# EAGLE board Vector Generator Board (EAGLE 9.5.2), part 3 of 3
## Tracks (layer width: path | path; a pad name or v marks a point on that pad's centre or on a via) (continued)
VRAM3  (via drill 0.35) (continued)
  Bottom 0.381: v4.36,171.92 4.65,171.92 4.65,170.46 P1.6 | v80.01,65.89 56.06,65.89 52.55,62.38 38.24,62.38 37.07,61.21 1G.5 | v80.89,94.81 79.43,96.27 79.43,97.73 75.34,97.73 v74.46,98.6 | v74.46,125.77 74.17,126.06 71.25,126.06 v67.45,129.86 | v67.45,153.52 67.16,153.81 60.44,153.81 58.1,156.15 38.24,156.15 37.07,157.31 1D.9 | v24.8,157.61 v10.49,157.61
VRAM4  (via drill 0.35)
  Top 0.381: v4.94,168.12 4.94,166.66 P1.7 4.94,166.37 7.28,164.03 9.61,164.03 v9.61,156.44 | v34.44,76.99 34.44,101.52 35.03,102.11 | 35.03,102.11 36.78,103.86 1F.2 | 52.84,151.18 52.84,133.07 52.26,132.49 52.26,98.02 v52.55,97.73 | 52.84,151.18 v52.84,235.01 | 35.03,102.11 v35.03,100.36 | v24.8,156.44 30.06,151.18 v31.23,151.18 | 52.84,151.18 v53.14,151.18
  Bottom 0.381: v4.94,168.12 4.94,166.66 P1.7 | v34.44,76.99 31.52,76.99 31.52,63.84 36.78,58.59 1G.6 | v52.84,235.01 38.24,235.01 37.07,236.18 1B.6 | v52.55,97.73 40.58,97.73 37.95,100.36 v35.03,100.36 | v24.8,156.44 v9.61,156.44 | v53.14,151.18 v31.23,151.18
VRAM5  (via drill 0.35)
  Top 0.381: v46.42,57.12 46.42,79.62 42.62,83.41 42.62,84.29 43.5,85.17 47.59,85.17 47.59,91.88 48.17,92.47 48.17,100.06 v47.88,100.36 | v32.11,233.55 31.81,233.26 31.81,225.37 v24.8,218.36 | v19.84,181.56 v19.84,216.03 | v4.94,164.03 4.94,162.57 P1.8 | v24.8,105.91 24.8,108.24 32.69,108.24 34.15,106.78 34.15,105.61 37.66,105.61 38.82,104.44 38.82,103.57 37.07,101.82 1F.3 | v11.07,105.91 10.78,106.2 10.78,140.08 12.24,141.54 v12.24,162.57
  Bottom 0.381: v46.42,57.12 38.24,57.12 37.07,55.96 1G.7 | v47.88,100.36 38.82,100.36 37.66,101.52 37.07,101.52 1F.3 | v32.11,233.55 36.78,233.55 1B.7 | v24.8,218.36 22.47,216.03 v19.84,216.03 | v19.84,181.56 11.07,172.8 10.2,172.8 9.61,172.21 9.61,164.03 | 9.61,162.57 9.61,164.03 | 9.61,162.57 4.94,162.57 P1.8 | 9.61,164.03 v4.94,164.03 | v11.07,105.91 v24.8,105.91 | 9.61,162.57 v12.24,162.57
VRAM6  (via drill 0.35)
  Top 0.381: v49.34,54.5 49.34,81.66 48.17,82.83 48.17,91.59 48.75,92.18 48.75,102.4 v48.46,102.69 | v35.03,204.93 35.03,213.98 37.36,216.32 37.36,218.36 35.03,220.7 35.03,229.17 36.78,230.92 1B.8 | v35.03,202.3 35.03,182.44 36.78,180.68 36.78,180.1 32.98,176.3 v32.98,164.03 32.98,163.16 28.6,158.78 v24.8,158.78 | v4.94,160.24 4.94,158.78 P1.9 | v58.69,102.69 58.98,102.98 58.98,116.42 58.1,117.3 58.1,121.97 58.98,122.85 58.98,123.72 58.1,124.6 55.18,124.6 v55.18,150.31 | v51.38,150.31 51.09,150.6 51.09,163.74 v51.38,164.03
  Bottom 0.381: v49.34,54.5 37.95,54.5 37.07,53.62 1G.8 | 1F.4 36.78,99.19 34.15,99.19 34.15,101.23 35.61,102.69 v48.46,102.69 v58.69,102.69 | v35.03,202.3 v35.03,204.93 | 4.94,158.78 v24.8,158.78 | 4.94,158.78 v4.94,160.24 | 4.94,158.78 P1.9 | v51.38,150.31 v55.18,150.31 | v32.98,164.03 v51.38,164.03
VRAM7  (via drill 0.35)
  Top 0.381: v4.94,156.15 4.94,154.69 P1.10 | 1G.9 36.78,50.99 35.03,52.74 35.03,72.9 36.78,74.65 36.78,81.66 35.03,83.41 35.03,94.51 36.78,96.27 1F.5 | v42.33,228.59 42.62,228.29 42.62,217.49 47.59,212.52 47.59,185.65 48.46,184.77 48.46,182.44 49.05,181.85 49.05,167.83 48.75,167.54 48.75,150.01 | 48.75,150.01 48.75,135.41 47,133.66 47,128.4 47.3,128.11 47.3,127.52 47,127.23 47,93.05 v47.3,92.76 | v24.8,154.39 25.97,154.39 30.35,150.01 v31.23,150.01 | 48.75,150.01 v48.46,150.01
  Bottom 0.381: v4.94,156.15 4.94,154.69 P1.10 4.94,154.39 v24.8,154.39 | v42.33,228.59 37.07,228.59 1B.9 | v47.3,92.76 40.58,92.76 37.07,96.27 1F.5 | v48.46,150.01 v31.23,150.01
VRAM8  (via drill 0.35)
  Top 0.381: 1F.6 39.41,96.56 39.41,106.78 35.9,110.29 20.13,110.29 v20.13,140.96 | v32.11,210.77 32.11,194.41 22.76,185.06 v22.76,181.56 | v19.84,143.59 v19.84,179.22 | v4.94,148.84 4.94,150.31 P1.11
  Bottom 0.381: 17.5,143.59 10.78,150.31 4.94,150.31 | 17.5,143.59 v20.13,140.96 | v32.11,210.77 36.78,210.77 1C.2 | v22.76,181.56 20.42,179.22 v19.84,179.22 | 17.5,143.59 v19.84,143.59 | 4.94,150.31 v4.94,148.84 | 4.94,150.31 P1.11
VRAM9  (via drill 0.35)
  Top 0.381: v31.23,111.16 28.89,113.5 21.3,113.5 v21.3,140.08 | v31.23,208.14 31.52,207.85 31.52,194.7 21.59,184.77 v21.59,181.56 | v21.01,143.59 v21.01,178.35 | v4.94,145.05 4.94,146.51 P1.12
  Bottom 0.381: v31.23,111.16 30.94,111.16 30.94,97.43 36.78,91.59 1F.7 | 21.01,140.08 14.58,140.08 9.61,145.05 | 9.61,145.05 8.15,146.51 4.94,146.51 P1.12 | v31.23,208.14 36.78,208.14 1C.3 | v21.59,181.56 20.13,180.1 19.55,180.1 18.96,179.51 18.96,178.35 v21.01,178.35 | 21.01,140.08 v21.01,143.59 | 21.01,140.08 v21.3,140.08 | 9.61,145.05 v4.94,145.05
VRAM10  (via drill 0.35)
  Top 0.381: v49.05,90.13 49.34,90.42 49.34,114.38 v49.05,114.67 | v31.23,115.25 23.05,123.43 v23.05,137.74 | 9.61,139.79 v9.61,137.74 | 9.61,139.79 6.98,142.42 4.94,142.42 P1.13 | v24.8,183.6 24.8,184.77 33.27,193.24 33.27,203.76 35.03,203.76 36.78,205.51 1C.4 | 11.37,142.42 11.37,141.54 9.61,139.79 | 11.37,142.42 v11.37,183.6 | 11.37,142.42 v11.07,142.42
  Bottom 0.381: v49.05,90.13 38.24,90.13 37.07,88.96 1F.8 | v49.05,114.67 48.75,114.96 31.52,114.96 v31.23,115.25 | v9.61,137.74 v23.05,137.74 | v11.37,183.6 v24.8,183.6 | v11.07,142.42 4.94,142.42 P1.13
VRAM11  (via drill 0.35)
  Top 0.381: v41.16,118.17 v41.16,86.34 | v31.23,118.17 23.93,125.48 v23.93,138.62 | v34.15,181.56 34.15,203.18 36.78,203.18 1C.5 | v31.23,179.22 24.8,172.8 23.93,172.8 v23.93,144.46 | v4.94,140.37 4.94,138.91 P1.14
  Bottom 0.381: v41.16,86.34 37.07,86.34 1F.9 | v31.23,118.17 v41.16,118.17 | 22.17,138.62 4.94,138.62 P1.14 4.94,138.91 v4.94,140.37 | 22.17,138.62 v23.93,138.62 | v34.15,181.56 31.81,179.22 v31.23,179.22 | v23.93,144.46 22.76,144.46 22.17,143.88 22.17,138.62
VRAMPC  (via drill 0.35)
  Top 0.381: v12.54,118.76 12.54,38.14 22.76,38.14 31.81,29.08 31.81,19.44 34.73,19.44 35.32,20.03 35.32,20.61 35.03,20.9 35.03,24.7 36.78,26.45 1H.3 | v4.94,120.51 4.94,119.05 P1.19
  Bottom 0.381: v12.54,118.76 4.94,118.76 P1.19 4.94,119.05 v4.94,120.51
XBRM1
  Top 0.381: 4A.13 105.42,277.95 115.65,267.73 115.65,251.08 120.03,246.7 120.03,240.56 118.28,238.81 5B.4
XBRM2
  Top 0.381: 4A.12 105.42,275.32 115.06,265.68 115.06,249.33 117.98,246.41 5B.1
XBRM3  (via drill 0.35)
  Top 0.381: v128.5,272.99 v128.5,241.44
  Bottom 0.381: v128.5,241.44 125.87,241.44 5B.14 | v128.5,272.99 105.42,272.99 4A.11
XBRM4  (via drill 0.35)
  Top 0.381: v103.38,245.24 103.67,245.53 103.67,268.9 105.13,270.36 4A.10 | v123.24,270.36 123.24,246.41 125.58,244.07 5B.15
  Bottom 0.381: v103.38,245.24 97.83,245.24 4B.1 | v123.24,270.36 105.42,270.36 4A.10
XBRM5
  Bottom 0.381: 4B.13 105.42,242.61 105.72,242.9 116.52,242.9 117.4,243.78 117.98,243.78 5B.2
XBRM6
  Bottom 0.381: 4B.12 105.42,240.27 106.01,240.86 117.69,240.86 117.98,241.15 5B.3
XBRM7  (via drill 0.35)
  Top 0.381: v102.5,274.15 102.5,240.27 105.13,237.64 4B.11
  Bottom 0.381: v102.5,274.15 117.98,274.15 5A.4
XBRM8  (via drill 0.35)
  Top 0.381: v103.38,209.6 103.67,209.89 103.67,215.74 106.59,218.66 106.59,228.88 107.17,229.46 107.17,232.97 105.42,234.72 4B.10 | v120.61,235.01 120.61,246.99 116.23,251.37 116.23,280 117.98,281.75 5A.1
  Bottom 0.381: v103.38,209.6 97.83,209.6 4C.1 | v120.61,235.01 105.42,235.01 4B.10
XBRM9  (via drill 0.35)
  Top 0.381: v99.87,207.26 99.87,266.85 100.17,267.14 v100.17,279.41
  Bottom 0.381: v99.87,207.26 105.13,207.26 4C.13 | v100.17,279.41 115.94,279.41 117.11,280.58 122.07,280.58 125.58,277.08 5A.14
XBRM10  (via drill 0.35)
  Top 0.381: v140.18,208.14 140.18,222.75 135.22,227.71 135.22,270.65 126.75,279.12 125.87,279.12 5A.15
  Bottom 0.381: v140.18,208.14 136.97,208.14 133.46,204.63 105.42,204.63 4C.12
XBRM11  (via drill 0.35)
  Top 0.381: v101.33,202.01 101.62,202.3 101.62,215.44 102.79,216.61 102.79,239.1 101.62,240.27 v101.62,277.08
  Bottom 0.381: v101.33,202.01 105.13,202.01 4C.11 | v101.62,277.08 115.94,277.08 117.98,279.12 5A.2
XBRM12  (via drill 0.35)
  Top 0.381: v112.43,198.79 112.73,199.09 112.73,215.44 113.02,215.74 113.02,223.62 | 113.02,223.62 113.02,239.4 111.56,240.86 111.56,268.31 108.05,271.82 103.67,271.82 103.67,278.83 104.25,279.41 108.34,279.41 v108.34,276.2 | v221.68,220.99 221.68,206.39 219.93,204.63 10C.3 | v99,223.62 v99,220.99 | 113.02,223.62 v112.73,223.62
  Bottom 0.381: 4C.10 106.01,198.79 v112.43,198.79 | v108.34,276.2 108.64,276.49 117.69,276.49 117.98,276.78 5A.3 | v221.68,220.99 159.46,220.99 159.17,221.28 142.81,221.28 142.52,220.99 112.14,220.99 111.85,221.28 102.21,221.28 101.92,220.99 v99,220.99 | v112.73,223.62 v99,223.62
XBRMCLK  (via drill 0.35)
  Top 0.381: 5B.9 125.87,228.88 127.62,230.63 127.62,262.18 125.87,263.93 5A.9 | v134.34,228.59 134.34,227.71 136.09,225.96 136.09,203.18 144.86,203.18 146.03,204.34 6C.12
  Bottom 0.381: v134.34,228.59 125.87,228.59 5B.9
XEND1  (via drill 0.35)
  Top 0.381: v58.98,263.06 58.98,248.16 57.23,246.41 2B.2 | v132.59,257.5 v132.59,208.43 | v186.63,257.5 186.63,263.93 8A.9 | v83.22,259.26 83.22,264.81 84.98,266.56 3A.10
  Bottom 0.381: 1B.19 44.67,246.41 56.93,246.41 2B.2 | v58.98,263.06 81.47,263.06 84.98,266.56 3A.10 | v132.59,208.43 125.87,208.43 5C.15 | v186.63,257.5 132.88,257.5 | v83.22,259.26 131.13,259.26 132.88,257.5 | 132.88,257.5 v132.59,257.5
XEND2  (via drill 0.35)
  Top 0.381: v77.67,255.75 77.67,263.93 3A.8 | 5C.1 118.28,210.77 121.49,207.56 123.83,207.56 123.83,234.72 121.2,237.35 v121.2,255.75 v121.2,265.39 | v59.86,255.75 59.86,246.7 57.23,244.07 2B.3
  Bottom 0.381: 1B.18 44.67,243.78 56.93,243.78 2B.3 | v121.2,255.75 v77.67,255.75 v59.86,255.75 | v121.2,265.39 146.9,265.39 148.07,266.56 167.35,266.56 168.81,268.02 185.46,268.02 186.63,269.19 8A.11
XEND3  (via drill 0.35)
  Top 0.381: v123.83,197.04 124.12,197.04 125.58,195.58 5C.10 | v91.4,220.99 v91.4,198.21 | v69.79,220.99 v69.79,239.98 69.79,271.82 v70.08,272.11 | 75.34,274.74 74.17,273.57 v74.17,272.11 | 75.34,274.74 77.38,276.78 3A.3 | v188.67,289.64 188.67,278.83 186.92,277.08 8A.14 | 75.34,274.74 v75.34,289.64
  Bottom 0.381: v123.83,197.04 107.47,197.04 106.3,198.21 v91.4,198.21 | v69.79,220.99 v91.4,220.99 | v69.79,239.98 58.39,239.98 57.23,241.15 2B.4 56.93,241.44 44.67,241.44 1B.17 | v70.08,272.11 v74.17,272.11 | v75.34,289.64 v188.67,289.64
XEND4  (via drill 0.35)
  Top 0.381: 74.46,290.51 64.82,290.51 64.82,282.63 63.94,281.75 61.61,281.75 61.61,243.19 57.23,238.81 2B.5 | 74.46,290.51 75.63,290.51 76.21,289.93 76.21,283.21 77.38,282.04 3A.1 | v170.56,278.54 v170.56,193.24 | v74.46,289.05 74.46,290.51 | v179.03,288.76 179.03,282.04 8A.1
  Bottom 0.381: 1B.16 44.67,238.81 56.93,238.81 2B.5 | v170.56,193.24 169.98,192.66 164.72,192.66 161.8,195.58 157.71,195.58 155.37,193.24 144.86,193.24 142.52,195.58 137.26,195.58 135.51,193.83 126.45,193.83 125.87,193.24 5C.9 | v170.56,278.54 173.77,281.75 179.03,281.75 8A.1 | v74.46,289.05 74.75,288.76 137.85,288.76 138.14,289.05 178.74,289.05 v179.03,288.76
XEND5  (via drill 0.35)
  Top 0.381: v114.48,173.97 114.48,195.29 v114.77,195.58 | v87.31,201.42 87.61,201.71 87.61,223.91 83.22,228.29 83.22,229.17 84.98,230.92 3B.10 | v172.31,254 v172.31,229.76 | v46.42,254 46.42,238.23 44.67,236.47 1B.15
  Bottom 0.381: v114.48,173.97 119.15,173.97 119.74,173.38 124.99,173.38 125.58,172.8 5D.15 | v114.77,195.58 92.86,195.58 87.31,201.13 v87.31,201.42 | v172.31,229.76 185.75,229.76 186.63,228.88 8B.9 | v172.31,254 172.02,253.71 46.71,253.71 v46.42,254 | 1B.15 44.67,236.18 56.93,236.18 2B.6 57.23,236.18 61.02,232.38 83.81,232.38 84.98,231.22 3B.10
XEND6  (via drill 0.35)
  Top 0.381: v58.98,227.42 58.98,231.8 57.23,233.55 2B.7 56.93,233.84 54.6,236.18 54.6,254 v54.01,254.58 | v116.81,191.49 116.81,176.59 117.98,175.43 5D.1 | v100.46,191.49 100.46,206.68 100.75,206.97 v100.75,216.03 | v77.67,216.03 77.67,228.59 3B.8 | v188.67,254.88 188.67,235.6 186.92,233.84 8B.11
  Bottom 0.381: 1B.14 44.67,233.84 56.93,233.84 2B.7 | v58.98,227.42 76.21,227.42 77.38,228.59 3B.8 | v100.46,191.49 v116.81,191.49 | v77.67,216.03 v100.75,216.03 | v188.67,254.88 122.37,254.88 121.78,254.29 54.31,254.29 v54.01,254.58
XEND7  (via drill 0.35)
  Top 0.381: v74.17,236.47 74.17,237.94 77.38,241.15 3B.3 | 2B.8 56.93,231.22 54.01,234.14 54.01,237.06 v53.72,237.35 53.14,237.94 v53.14,255.46 | v88.48,174.84 88.19,175.13 88.19,177.18 86.73,178.64 86.73,192.37 87.02,192.66 87.02,195.87 85.85,197.04 83.22,197.04 83.22,206.1 84.1,206.97 87.02,206.97 87.02,223.62 80.3,230.34 v80.3,237.35 | v184.87,255.75 184.87,243.19 186.63,241.44 8B.14
  Bottom 0.381: 1B.13 44.67,231.22 56.93,231.22 2B.8 | v74.17,236.47 73.29,237.35 v53.72,237.35 | v88.48,174.84 89.94,174.84 94.62,170.17 99,170.17 103.96,165.2 106.3,165.2 107.47,164.03 121.78,164.03 125.58,160.24 5D.10 | v80.3,237.35 80.3,240.27 78.55,240.27 77.67,241.15 3B.3 | v184.87,255.75 184.58,255.46 122.07,255.46 121.49,254.88 54.89,254.88 54.31,255.46 v53.14,255.46
XEND8  (via drill 0.35)
  Top 0.381: v108.05,158.78 108.34,159.07 108.34,182.14 108.05,182.44 108.05,189.74 108.93,190.61 v108.93,243.78 v108.93,257.5 | v130.25,257.5 v130.25,244.94 | v79.43,229.76 79.43,244.36 77.67,246.11 3B.1
  Bottom 0.381: 1B.12 44.67,228.59 56.93,228.59 2B.9 57.23,228.88 58.1,229.76 v79.43,229.76 | v108.05,158.78 119.15,158.78 119.74,158.19 124.99,158.19 125.58,157.61 5D.9 | v108.93,243.78 87.61,243.78 86.14,245.24 78.55,245.24 77.67,246.11 3B.1 | v130.25,244.94 147.19,244.94 148.36,243.78 176.69,243.78 179.03,246.11 8B.1 | v108.93,257.5 v130.25,257.5
XEND9  (via drill 0.35)
  Top 0.381: 1C.19 44.67,210.77 46.42,209.02 v46.42,182.44 v46.42,175.43 46.42,161.4 43.5,161.4 42.04,159.94 42.04,153.22 42.33,152.93 v42.33,144.46 | v124.12,143.59 123.83,143.29 123.83,138.91 125.58,137.16 5E.15 | v83.22,182.14 83.22,193.83 84.98,195.58 3C.10 | v186.63,178.93 186.63,192.95 8C.9
  Bottom 0.381: v46.42,175.43 56.93,175.43 2D.2 | v124.12,143.59 123.83,143.29 43.5,143.29 v42.33,144.46 | v46.42,182.44 48.46,182.44 48.75,182.14 v83.22,182.14 83.81,182.73 89.06,182.73 90.53,181.27 126.16,181.27 128.5,178.93 v186.63,178.93
XEND10  (via drill 0.35)
  Top 0.381: v114.77,170.17 114.77,158.48 118.28,154.98 118.28,139.79 5E.1 | v77.67,178.05 77.67,192.95 3C.8 | 2D.3 59.86,175.43 v59.86,192.95 | v160.05,192.07 156.54,188.57 156.54,188.28 154.79,186.53 v153.91,186.53 | v122.66,171.34 v122.66,184.77
  Bottom 0.381: v77.67,178.05 91.69,178.05 94.32,175.43 98.7,175.43 103.96,170.17 v114.77,170.17 115.94,171.34 v122.66,171.34 | 3C.8 77.38,192.95 v59.86,192.95 59.86,193.83 58.1,195.58 56.06,195.58 49.92,201.71 42.62,201.71 42.62,206.39 44.37,208.14 1C.18 | v160.05,192.07 170.56,192.07 172.61,194.12 182.83,194.12 186.63,197.92 8C.11 | v153.91,186.53 130.84,186.53 129.08,184.77 v122.66,184.77
XEND11  (via drill 0.35)
  Top 0.381: v55.47,205.51 55.18,205.22 55.18,172.21 56.93,170.46 2D.4 | v130.25,124.89 130.54,125.18 130.54,138.33 v130.25,138.62 129.96,138.91 129.96,163.16 v130.25,163.45 | v106.59,140.96 105.13,142.42 v105.13,150.89 | v80.89,150.89 81.18,151.18 81.18,172.5 82.35,173.67 82.35,180.97 79.43,183.9 79.43,203.76 77.67,205.51 3C.3 77.38,205.8 72.12,205.8 v69.79,208.14 | v189.55,178.64 v189.55,205.51 | v146.03,177.18 146.03,167.54 142.81,164.32 v142.81,163.45
  Bottom 0.381: 1C.17 44.67,205.51 v55.47,205.51 55.77,205.8 61.32,205.8 63.65,208.14 v69.79,208.14 | 5E.10 126.16,124.89 v130.25,124.89 | v130.25,138.62 121.49,138.62 119.15,140.96 v106.59,140.96 | v80.89,150.89 v105.13,150.89 | v189.55,205.51 186.92,205.51 8C.14 | v189.55,178.64 188.09,177.18 v146.03,177.18 | v130.25,163.45 v142.81,163.45
XEND12  (via drill 0.35)
  Top 0.381: 54.6,167.83 53.72,167.83 v53.72,203.18 v53.72,219.24 | 54.6,167.83 56.93,167.83 2D.5 | v125.58,117.88 125.58,121.68 5E.9 | v42.33,118.17 42.04,118.47 v42.04,132.19 | v56.06,139.79 56.06,150.89 54.6,152.35 54.6,167.83 | v76.8,219.24 76.8,211.65 77.38,211.06 3C.1
  Bottom 0.381: v53.72,203.18 44.67,203.18 1C.16 | v125.58,117.88 125.28,118.17 60.44,118.17 60.15,118.47 42.62,118.47 v42.33,118.17 | v42.04,132.19 46.13,132.19 47.59,133.66 49.92,133.66 v56.06,139.79 | v53.72,219.24 v76.8,219.24 | 8C.1 179.03,210.77 176.69,208.43 162.67,208.43 160.34,210.77 149.53,210.77 147.19,208.43 141.94,208.43 139.6,210.77 131.13,210.77 129.96,209.6 110.39,209.6 106.59,205.8 92.28,205.8 91.69,206.39 89.36,206.39 86.14,209.6 78.84,209.6 77.67,210.77 3C.1
XOUT
  Top 0.381: VR2.3 198.31,128.11 198.31,125.77 VR2.2
  Bottom 0.381: C43.1 188.09,125.77 198.02,125.77 VR2.2 198.31,125.77 205.61,125.77 IC10.1 205.91,125.48 209.41,125.48 212.92,121.97 216.13,121.97 231.32,106.78 235.7,106.78 241.25,101.23 X1.5
XRATE  (via drill 0.35)
  Top 0.381: v113.6,138.33 113.31,138.62 113.31,164.91 112.14,166.08 v112.14,169 | v128.5,205.51 128.21,205.22 128.21,184.48 127.62,183.9 127.62,172.21 125.87,170.46 5D.14 | 5B.6 118.28,233.55 120.32,231.51 120.32,215.44 116.23,211.35 116.23,207.85 117.11,206.97 120.32,206.97 121.49,205.8 125.58,205.8 5C.14
  Bottom 0.381: v113.6,138.33 119.15,138.33 119.44,138.04 122.37,138.04 125.58,134.82 5E.14 | v112.14,169 120.03,169 121.2,170.17 125.58,170.17 5D.14 | v128.5,205.51 125.87,205.51 5C.14
YBRM1  (via drill 0.35)
  Top 0.381: v87.61,178.93 87.61,200.55 88.19,201.13 88.19,211.65 89.36,212.81 v89.36,256.63 | v140.18,256.63 140.18,240.56 138.43,238.81 6B.4
  Bottom 0.381: v87.61,178.93 103.67,178.93 103.67,173.09 105.13,171.63 4D.13 | v140.18,256.63 v89.36,256.63
YBRM2  (via drill 0.35)
  Top 0.381: v108.05,245.24 108.05,229.46 107.17,228.59 107.17,193.83 106.88,193.53 106.88,176.89 107.17,176.59 107.17,170.75 105.42,169 4D.12
  Bottom 0.381: v108.05,245.24 129.38,245.24 130.25,246.11 138.43,246.11 6B.1
YBRM3  (via drill 0.35)
  Top 0.381: v113.02,183.9 v113.02,166.37 | v111.56,184.77 111.56,199.09 112.14,199.67 v112.14,216.03 | v127.04,216.03 128.5,217.49 v128.5,239.1
  Bottom 0.381: v113.02,166.37 4D.11 | v113.02,183.9 112.14,184.77 v111.56,184.77 | v127.04,216.03 v112.14,216.03 | v128.5,239.1 128.79,239.4 136.68,239.4 137.26,239.98 140.47,239.98 141.64,241.15 146.03,241.15 6B.14
YBRM4  (via drill 0.35)
  Top 0.381: v100.46,163.74 100.46,159.07 99.29,157.9 99.29,140.08 97.83,138.62 4E.1 | v130.84,218.36 v130.84,242.61 | v108.05,218.36 107.76,218.07 107.76,190.32 107.47,190.03 107.47,177.18 107.76,176.89 107.76,166.37 105.42,164.03 4D.10
  Bottom 0.381: v100.46,163.74 105.13,163.74 4D.10 | v130.84,242.61 144.86,242.61 146.03,243.78 6B.15 | v130.84,218.36 130.54,218.07 122.66,218.07 122.37,218.36 v108.05,218.36
YBRM5  (via drill 0.35)
  Top 0.381: v102.79,136.87 103.09,137.16 103.09,174.55 102.21,175.43 v101.92,175.43 | v94.62,176.3 90.23,176.3 90.23,190.32 89.36,191.2 89.36,191.78 92.28,194.7 92.28,229.76 93.45,230.92 v93.45,241.44
  Bottom 0.381: v102.79,136.87 104.25,136.87 105.13,135.99 4E.13 | v101.92,175.43 101.04,176.3 v94.62,176.3 | v93.45,241.44 115.94,241.44 117.11,242.61 129.67,242.61 130.84,243.78 138.43,243.78 6B.2
YBRM6  (via drill 0.35)
  Top 0.381: v101.33,135.99 101.33,152.64 101.92,153.22 101.92,173.38 101.04,174.26 101.04,183.31 101.33,183.6 v101.33,192.37 | v113.02,192.37 113.31,192.66 113.31,215.15 113.6,215.44 v113.6,239.98
  Bottom 0.381: v101.33,135.99 102.5,135.99 105.13,133.36 4E.12 | v113.02,192.37 v101.33,192.37 | v113.6,239.98 136.38,239.98 137.55,241.15 138.43,241.15 6B.3
YBRM7  (via drill 0.35)
  Top 0.381: v110.97,130.73 110.97,145.05 v107.47,148.55 | v109.51,148.84 109.51,181.56 113.89,185.94 113.89,214.86 119.44,220.41 v119.44,227.42 | v136.68,227.42 136.68,272.4 138.43,274.15 6A.4
  Bottom 0.381: v110.97,130.73 105.42,130.73 4E.11 | v107.47,148.55 107.76,148.84 v109.51,148.84 | v136.68,227.42 v119.44,227.42
YBRM8  (via drill 0.35)
  Top 0.381: v98.12,114.67 98.12,103.28 97.83,102.98 4F.1 | 103.67,126.64 v103.67,114.67 | 103.67,126.64 105.13,128.11 4E.10 | v138.43,288.18 6A.1 | v50.22,288.18 50.22,185.36 v50.51,185.06 | v100.46,183.9 100.46,164.91 101.33,164.03 101.33,153.81 v101.04,153.52 | v103.96,153.52 103.67,153.22 103.67,126.64
  Bottom 0.381: v103.67,114.67 v98.12,114.67 | v50.22,288.18 v138.43,288.18 | v50.51,185.06 51.97,183.6 82.93,183.6 83.52,184.19 100.17,184.19 v100.46,183.9 | v103.96,153.52 v101.04,153.52
YBRM9  (via drill 0.35)
  Top 0.381: v90.23,123.72 v90.23,104.74 | v88.19,154.69 v88.19,131.9 | v88.19,158.48 87.9,158.78 87.9,166.95 87.61,167.25 87.61,176.59 81.76,182.44 v81.76,204.63 | v72.42,258.38 v72.42,210.48 | v130.84,272.99 v130.84,258.38
  Bottom 0.381: v90.23,104.74 98.12,104.74 101.62,101.23 104.25,101.23 105.13,100.36 4F.13 | v90.23,123.72 90.23,124.31 86.14,128.4 83.81,128.4 83.22,128.98 83.22,131.03 87.31,131.03 v88.19,131.9 | v88.19,158.48 v88.19,154.69 | v81.76,204.63 76.21,204.63 72.42,208.43 v72.42,210.48 | v130.84,258.38 v72.42,258.38 | v130.84,272.99 146.9,272.99 147.78,273.86 147.78,276.78 146.32,276.78 6A.14
YBRM10  (via drill 0.35)
  Top 0.381: v114.48,101.23 114.19,101.52 114.19,126.35 v114.48,126.64 | v113.6,133.66 116.23,136.28 116.23,146.8 116.52,147.09 v116.52,151.18 | v127.33,151.18 127.62,151.47 127.62,171.34 128.21,171.92 128.21,183.6 130.25,185.65 130.25,197.33 130.84,197.92 v130.84,214.27 | v144.86,214.27 148.36,217.78 148.36,277.08 146.32,279.12 6A.15
  Bottom 0.381: v114.48,101.23 111.85,98.6 106.01,98.6 105.42,98.02 4F.12 | v114.48,126.64 114.19,126.94 104.55,126.94 103.67,127.81 103.67,132.19 111.27,132.19 112.73,133.66 v113.6,133.66 | v127.33,151.18 v116.52,151.18 | v144.86,214.27 v130.84,214.27
YBRM11  (via drill 0.35)
  Top 0.381: v130.54,100.36 130.84,100.65 130.84,108.24 130.25,108.83 130.25,123.72 131.13,124.6 131.13,139.79 130.54,140.37 130.54,162.28 v130.84,162.57 | v134.05,164.32 v134.05,162.57 | v133.46,168.71 133.46,271.53 128.5,276.49 v128.21,276.49
  Bottom 0.381: v130.54,100.36 117.11,100.36 114.77,98.02 108.05,98.02 105.42,95.39 4F.11 | v134.05,162.57 v130.84,162.57 | v134.05,164.32 133.76,164.03 131.42,164.03 130.84,164.62 130.84,168.71 v133.46,168.71 | v128.21,276.49 130.84,279.12 138.43,279.12 6A.2
YBRM12  (via drill 0.35)
  Top 0.381: v128.5,93.34 128.21,93.64 128.21,114.96 129.38,116.13 129.38,129.56 v129.67,129.86 | v133.17,130.15 133.17,138.91 133.46,139.2 133.46,145.92 134.63,147.09 v134.63,153.81 | 214.38,201.71 v214.38,164.91 | 214.38,201.71 219.63,206.97 10C.2 | v136.68,287.01 136.68,278.83 138.43,277.08 6A.3 | v211.46,287.01 211.46,204.63 214.38,201.71
  Bottom 0.381: v128.5,93.34 127.91,92.76 105.42,92.76 4F.10 | v129.67,129.86 129.96,130.15 v133.17,130.15 | v134.63,153.81 134.63,155.27 142.52,155.27 152.16,164.91 v214.38,164.91 | v211.46,287.01 v136.68,287.01
YBRMCLK  (via drill 0.35)
  Top 0.381: v135.22,216.03 135.22,200.25 138.43,197.04 6C.6 | v144.86,216.03 146.03,217.19 146.03,228.59 6B.9 146.32,228.88 147.78,230.34 147.78,262.47 146.32,263.93 6A.9
  Bottom 0.381: v144.86,216.03 v135.22,216.03
YEND1  (via drill 0.35)
  Top 0.381: v73,166.37 v73,161.7 | v122.37,121.39 122.37,119.63 123.83,118.17 123.83,103.57 125.58,101.82 5F.15 | v82.06,140.96 82.35,141.25 82.35,157.31 84.98,159.94 3D.10 | 9A.9 202.98,260.13 202.98,223.62 202.11,222.75 v202.11,220.12 | v65.41,218.36 62.78,215.74 v62.78,167.25
  Bottom 0.381: 1D.15 44.67,165.2 56.93,165.2 2D.6 57.23,165.2 58.39,166.37 62.78,166.37 | v73,161.7 74.75,161.7 75.04,161.4 83.81,161.4 84.98,160.24 3D.10 | 62.78,166.37 v73,166.37 | v122.37,121.39 120.9,121.39 119.15,123.14 107.76,123.14 106.3,124.6 104.25,124.6 103.09,125.77 103.09,134.53 92.57,134.53 86.14,140.96 v82.06,140.96 | v202.11,220.12 201.82,220.41 159.17,220.41 158.88,220.7 143.1,220.7 142.81,220.41 111.85,220.41 111.56,220.7 102.5,220.7 100.17,218.36 v65.41,218.36 | 62.78,166.37 v62.78,167.25
YEND2  (via drill 0.35)
  Top 0.381: 124.12,128.4 124.12,128.69 123.53,129.27 121.78,129.27 121.78,128.98 121.2,128.4 116.81,128.4 114.19,131.03 112.43,131.03 112.43,131.32 112.14,131.61 112.14,147.68 v111.85,147.97 | 124.12,128.4 124.12,128.11 120.61,124.6 120.61,122.26 119.15,120.8 119.15,105.03 118.28,104.15 5F.1 | v76.8,147.97 77.38,148.55 77.38,157.31 3D.8 | v212.33,173.97 212.33,201.13 210.87,202.59 210.87,265.39 207.07,269.19 9A.11 | v128.5,170.46 128.21,170.17 128.21,129.86 126.75,128.4 124.12,128.4 | v41.45,148.26 41.45,162.28 44.37,162.28 1D.14
  Bottom 0.381: 1D.14 44.67,162.57 56.93,162.57 2D.7 | v111.85,147.97 111.56,147.68 77.09,147.68 v76.8,147.97 56.64,147.97 56.35,148.26 v41.45,148.26 | v212.33,173.97 135.51,173.97 132.88,171.34 130.54,171.34 129.67,170.46 v128.5,170.46
YEND3  (via drill 0.35)
  Top 0.381: v113.02,90.13 113.02,127.52 v113.31,127.81 | v107.47,127.81 107.47,143.88 v107.17,144.17 | v59.56,144.17 59.56,158.48 58.1,159.94 57.23,159.94 2D.8 | v152.16,229.76 v152.16,274.45 | v96.08,228.59 96.08,206.39 96.66,205.8 99.58,205.8 99.58,204.05 98.7,203.18 96.08,203.18 96.08,201.42 94.62,199.96 94.62,180.39 v91.4,177.18
  Bottom 0.381: 1D.13 44.67,160.24 56.93,160.24 2D.8 57.23,160.24 61.02,164.03 79.43,164.03 79.43,168.42 77.67,170.17 3D.3 77.67,170.46 79.43,170.46 79.43,173.09 82.93,176.59 90.82,176.59 v91.4,177.18 | v113.02,90.13 119.15,90.13 119.74,89.55 124.99,89.55 125.58,88.96 5F.10 | v107.47,127.81 v113.31,127.81 | v59.56,144.17 v107.17,144.17 | v152.16,274.45 167.64,274.45 169.39,276.2 173.48,276.2 177.86,280.58 208.83,280.58 208.83,278.83 207.07,277.08 9A.14 | v152.16,229.76 107.47,229.76 106.3,228.59 v96.08,228.59
YEND4  (via drill 0.35)
  Top 0.381: v132,110.87 v132,86.63 | v108.34,114.08 108.34,128.11 108.05,128.4 v108.05,145.63 | v46.42,145.92 46.42,155.56 44.67,157.31 1D.12 | 76.8,174.55 75.34,173.09 v75.34,162.57 | 76.8,174.55 77.38,175.13 3D.1 | v194.51,270.36 194.51,277.08 199.19,281.75 9A.1 | v110.68,268.02 110.68,220.41 110.39,220.12 110.39,201.13 110.68,200.84 110.68,199.96 109.8,199.09 v109.8,185.06 | 76.8,174.55 v76.8,185.06
  Bottom 0.381: 1D.12 44.67,157.61 56.93,157.61 2D.9 57.23,157.61 58.1,157.61 61.61,161.11 65.7,161.11 67.16,162.57 v75.34,162.57 | v132,86.63 125.87,86.63 5F.9 | v132,110.87 131.71,111.16 111.27,111.16 v108.34,114.08 | v108.05,145.63 107.76,145.92 v46.42,145.92 | v194.51,270.36 168.52,270.36 167.35,269.19 148.36,269.19 147.19,268.02 v110.68,268.02 | v109.8,185.06 109.51,185.36 77.09,185.36 v76.8,185.06
YEND5  (via drill 0.35)
  Top 0.381: v52.84,83.41 v52.84,77.57 | v54.6,84.87 54.6,92.18 54.01,92.76 54.01,103.86 v53.72,104.15 | v62.19,104.15 v62.19,120.8 | v204.15,163.74 204.15,210.19 205.61,211.65 205.61,227.42 206.78,228.59 9B.9 | v148.65,153.22 148.65,144.46 149.24,143.88 149.24,137.45 v148.95,137.16 | v136.97,137.16 136.68,136.87 136.68,124.02 136.97,123.72 136.97,121.09 135.8,119.93 135.8,114.96 133.46,112.62 v133.46,77.57
  Bottom 0.381: 1F.19 44.67,104.15 v53.72,104.15 56.93,104.15 2F.2 57.23,104.15 v62.19,104.15 | 5G.15 131.42,71.73 131.42,77.57 | 131.42,77.57 114.19,77.57 113.89,77.28 84.39,77.28 83.81,77.86 53.14,77.86 v52.84,77.57 | v52.84,83.41 54.31,84.87 v54.6,84.87 | v62.19,120.8 81.47,120.8 84.98,124.31 3E.10 | v204.15,163.74 185.46,163.74 177.28,155.56 163.26,155.56 160.92,153.22 v148.65,153.22 | v136.97,137.16 v148.95,137.16 | 131.42,77.57 v133.46,77.57
YEND6  (via drill 0.35)
  Top 0.381: v108.05,111.75 v108.05,68.81 | v77.67,112.62 77.67,121.68 3E.8 | v203.28,183.9 203.28,210.19 205.03,211.94 205.03,231.8 206.78,233.55 9B.11 | v148.65,181.56 148.65,166.08 147.48,164.91 145.15,164.91 145.15,151.76 144.56,151.18 v144.56,145.05 | v123.24,145.05 122.95,144.75 122.95,131.32 v120.9,129.27 | v115.94,115.84 v115.94,128.11 | v58.98,121.68 58.98,117.3 59.56,116.71 59.56,101.82 57.23,101.82 2F.3
  Bottom 0.381: 1F.18 44.67,101.82 56.93,101.82 2F.3 | v108.05,68.81 117.98,68.81 5G.1 | v108.05,111.75 107.17,112.62 104.55,112.62 | v77.67,112.62 104.55,112.62 | v203.28,183.9 202.4,183.02 173.77,183.02 172.31,181.56 v148.65,181.56 | v123.24,145.05 v144.56,145.05 | v120.9,129.27 119.74,128.11 v115.94,128.11 | v115.94,115.84 105.13,115.84 104.55,115.25 104.55,112.62 | v58.98,121.68 77.38,121.68 3E.8
YEND7  (via drill 0.35)
  Top 0.381: v74.17,85.46 v74.17,55.66 | 46.42,97.14 v46.42,87.5 | 46.42,97.14 44.67,98.9 1F.17 | v70.08,134.24 70.08,134.53 77.38,134.53 3E.3 | 46.42,97.14 v46.42,127.81 | v196.27,239.98 196.27,179.22 202.11,173.38 202.11,161.11 v201.82,160.82 | v123.53,161.11 v123.53,146.22 | v92.57,160.24 82.93,150.6 v82.93,138.33
  Bottom 0.381: 1F.17 44.67,99.19 56.93,99.19 2F.4 | v74.17,55.66 86.44,55.66 88.77,53.33 106.3,53.33 107.47,54.5 119.15,54.5 119.44,54.2 124.99,54.2 125.58,53.62 5G.10 | v74.17,85.46 72.12,87.5 v46.42,87.5 | v70.08,134.24 69.79,134.53 63.36,134.53 58.39,129.56 48.17,129.56 v46.42,127.81 | v196.27,239.98 205.61,239.98 206.78,241.15 9B.14 | v201.82,160.82 195.1,160.82 188.09,153.81 166.47,153.81 158.88,146.22 v123.53,146.22 | v123.53,161.11 107.47,161.11 106.59,160.24 v92.57,160.24 | v82.93,138.33 79.43,134.82 77.67,134.82 3E.3
YEND8  (via drill 0.35)
  Top 0.381: v80.59,44.86 75.04,44.86 75.04,55.96 74.75,56.25 74.75,72.02 79.43,76.69 v79.43,91.3 | v67.45,123.14 67.45,98.9 v67.16,98.6 | 3E.1 77.38,139.5 75.63,137.74 75.63,136.58 76.5,135.7 81.47,135.7 81.47,129.27 v82.06,128.69 82.06,128.4 90.53,128.4 93.15,131.03 v93.15,157.61 | v151.28,218.36 v151.28,241.15 | v134.34,191.78 v134.34,218.36 | v124.41,178.93 v124.41,191.78 | v112.14,178.93 112.14,170.17 111.27,169.29 111.27,157.9 v111.56,157.61
  Bottom 0.381: 1F.16 44.67,96.56 56.93,96.56 2F.5 57.23,96.56 58.39,97.73 67.16,97.73 | v80.59,44.86 80.89,45.15 82.35,45.15 82.64,44.86 117.4,44.86 119.15,46.61 121.49,46.61 125.58,50.7 5G.9 | v79.43,91.3 79.43,92.76 72.71,92.76 67.74,97.73 67.16,97.73 | v82.06,128.69 82.06,123.14 v67.45,123.14 | 67.16,97.73 v67.16,98.6 | v151.28,241.15 167.64,241.15 168.81,239.98 187.8,239.98 191.3,243.48 196.56,243.48 199.19,246.11 9B.1 | v134.34,218.36 v151.28,218.36 | v124.41,191.78 v134.34,191.78 | v112.14,178.93 v124.41,178.93 | v93.15,157.61 v111.56,157.61
YEND9  (via drill 0.35)
  Top 0.381: 2F.6 57.23,93.93 v59.27,95.97 60.15,96.85 60.15,117.3 v59.86,117.59 | v131.42,30.54 131.42,34.34 130.25,35.51 130.25,76.4 v130.54,76.69 | v83.52,76.99 83.22,77.28 83.22,86.92 84.98,88.67 3F.10 | v199.48,140.67 199.19,140.96 199.19,148.84 200.94,148.84 207.37,155.27 207.37,192.66 207.07,192.95 9C.9 | v135.8,141.83 134.92,140.96 134.92,130.73 133.46,129.27 v133.46,117
  Bottom 0.381: 1F.15 44.67,93.93 56.93,93.93 2F.6 | v59.27,95.97 59.56,95.97 62.78,92.76 71.83,92.76 74.46,90.13 83.81,90.13 84.98,88.96 3F.10 | v131.42,30.54 125.87,30.54 5H.15 | v130.54,76.69 130.25,76.99 114.48,76.99 114.19,76.69 83.81,76.69 v83.52,76.99 | v199.48,140.67 198.6,141.54 136.09,141.54 v135.8,141.83 | v133.46,117 101.33,117 100.75,117.59 v59.86,117.59
YEND10  (via drill 0.35)
  Top 0.381: v127.04,34.34 128.21,35.51 v128.21,76.11 | v77.67,76.11 77.67,86.34 3F.8 | v208.83,174.84 208.83,196.16 207.07,197.92 9C.11 | v138.43,166.66 v138.43,174.84 | v54.31,149.43 54.6,149.14 54.6,108.83 55.18,108.24 55.18,93.34 56.93,91.59 2F.7
  Bottom 0.381: 1F.14 44.67,91.59 56.93,91.59 2F.7 57.23,91.3 58.98,91.3 60.15,90.13 65.7,90.13 66.28,89.55 74.46,89.55 77.38,86.63 3F.8 | v127.04,34.34 119.44,34.34 118.28,33.17 5H.1 | v77.67,76.11 v128.21,76.11 | v138.43,174.84 v208.83,174.84 | v138.43,166.66 138.43,164.03 142.23,164.03 142.52,164.32 143.1,164.32 143.69,163.74 143.69,158.78 136.09,158.78 127.62,150.31 115.35,150.31 115.06,150.6 106.01,150.6 105.13,149.72 55.77,149.72 55.47,149.43 v54.31,149.43
YEND11  (via drill 0.35)
  Top 0.381: v113.89,19.15 111.56,21.49 111.56,66.47 110.68,67.35 v110.68,99.48 | v209.7,161.7 209.7,202.88 207.07,205.51 9C.14 | v165.59,135.7 v165.59,154.1 | v134.34,117.88 v134.34,128.98 | v127.04,117.88 127.04,105.03 127.62,104.44 127.62,102.98 v127.33,102.69 | 2F.8 57.23,88.96 60.15,88.96 60.15,93.34 62.78,95.97 62.78,96.85 63.65,97.73 77.38,97.73 77.38,98.9 3F.3
  Bottom 0.381: 1F.13 44.67,88.96 56.93,88.96 2F.8 | v113.89,19.15 119.15,19.15 119.74,18.57 124.99,18.57 125.58,17.98 5H.10 | 3F.3 77.38,99.19 75.04,99.19 75.04,105.03 75.92,105.91 87.9,105.91 94.62,99.19 110.39,99.19 v110.68,99.48 113.89,102.69 v127.33,102.69 | v209.7,161.7 195.1,161.7 187.8,154.39 165.89,154.39 v165.59,154.1 | v165.59,135.7 146.61,135.7 139.89,128.98 v134.34,128.98 | v127.04,117.88 v134.34,117.88
YEND12  (via drill 0.35)
  Top 0.381: v58.98,82.54 58.98,84.58 57.23,86.34 2F.9 | v115.35,91.3 115.35,6.59 117.11,6.59 125.58,15.06 5H.9 | v191.3,178.64 v191.3,210.77 | v158.29,176.3 158,176.01 158,173.09 156.25,171.34 156.25,164.91 149.53,158.19 v149.53,147.97 | v115.65,147.38 115.65,139.5 v115.35,139.2 | v109.51,139.2 109.51,115.25 v110.68,114.08 | v115.94,114.08 115.94,101.52 114.48,100.06 v114.48,93.93
  Bottom 0.381: 1F.12 44.67,86.34 56.93,86.34 2F.9 | 83.22,95.1 83.22,92.76 86.14,92.76 87.02,91.88 87.02,87.5 80.89,87.5 75.92,82.54 v58.98,82.54 | 83.22,95.1 83.22,98.31 77.67,103.86 3F.1 | v115.35,91.3 115.06,91.59 103.67,91.59 | 103.67,91.59 90.23,91.59 86.73,95.1 83.22,95.1 | v191.3,210.77 199.19,210.77 9C.1 | v191.3,178.64 188.96,176.3 v158.29,176.3 | v149.53,147.97 134.34,147.97 133.76,148.55 118.28,148.55 117.11,147.38 v115.65,147.38 | v109.51,139.2 v115.35,139.2 | v115.94,114.08 v110.68,114.08 | v114.48,93.93 104.25,93.93 103.67,93.34 103.67,91.59
YOUT
  Top 0.381: VR4.3 198.31,64.72 198.31,62.38 VR4.2
  Bottom 0.381: C59.1 188.09,63.26 188.96,62.38 198.02,62.38 VR4.2 198.31,62.38 205.61,62.38 IC15.1 | X1.3 241.54,93.05 244.46,90.13 244.46,65.01 198.31,65.01 VR4.3
YRATE  (via drill 0.35)
  Top 0.381: 127.62,61.51 127.62,50.41 123.83,46.61 123.83,29.96 125.58,28.21 5H.14 | 127.62,61.51 125.87,63.26 5G.14 | 127.62,61.51 127.62,69.1 127.33,69.39 127.33,76.4 127.62,76.69 v127.62,85.46 127.62,97.14 125.87,98.9 5F.14 | v140.47,239.1 140.47,235.89 138.43,233.84 6B.6 | v176.11,238.81 176.11,190.32 176.99,189.45 v176.99,179.81 | v205.91,179.81 205.61,179.51 205.61,154.39 200.65,149.43 198.6,149.43 v198.6,137.45 | v138.43,126.64 v138.43,138.04 | v135.22,126.64 135.22,115.25 132.88,112.92 132.88,85.75 v132.59,85.46
  Bottom 0.381: v140.47,239.1 141.35,239.98 156.54,239.98 157.71,238.81 v176.11,238.81 | v205.91,179.81 v176.99,179.81 | v198.6,137.45 161.51,137.45 160.63,138.33 138.72,138.33 v138.43,138.04 | v135.22,126.64 v138.43,126.64 | v127.62,85.46 v132.59,85.46
ZOUT  (via drill 0.35)
  Top 0.381: R26.2 132.3,172.5 132.3,167.83 T2.3 132,167.54 130.84,166.37 130.84,164.03 131.71,163.16 131.71,162.28 131.13,161.7 131.13,140.96 v131.42,140.67 | v237.74,111.45 237.74,88.96 241.25,85.46 X1.1
  Bottom 0.381: v131.42,140.67 131.71,140.37 195.97,140.37 197.14,139.2 198.9,139.2 211.16,126.94 217,126.94 231.03,112.92 236.28,112.92 v237.74,111.45

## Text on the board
Top: 1 | 2 | 3 | 4 | 5 | 6 | 7 | 8 | 9 | Note: The analog circuits on this board / were NOT designed by Kincaid Arcade; / they were copied from the Atari Asteroids / Deluxe Manual. This project is intended / ONLY as a hobbyist's attempt to make a / vector arcade game, and neither Alexander / Haley nor Kincaid Arcade claim copyright or / ownership on any of the analog circuits. | Kincaid Arcade | A | Vector Generator | Board REV-A | (c) Kincaid Arcade | 2/9/2020 | KincaidArcade.com | Digital Circuits | Designed By: | B | Alexander K. Haley | (A 16 Year Old!) | +5V | C | Power Supply | +5V / DAC | +15V | -15V | D | X Analog Circuitry | X Gain | E | X Center | F | Y Analog Circuitry | Y Gain | G | Y Center | H | The manufacture of this board / for resale at a profit is strictly / prohibited.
